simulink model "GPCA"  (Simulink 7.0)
settings: Solver=ode45  StartTime=0.0  StopTime=inf  RelTol=1e-3
PreLoadFcn:
  | GPCA_Bus_Def
InitFcn:
  | script
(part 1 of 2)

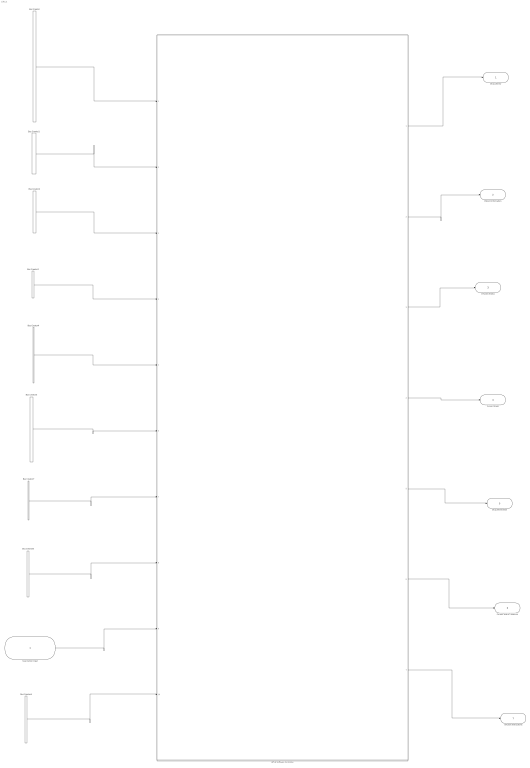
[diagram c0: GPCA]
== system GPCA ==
  User Action Input : Inport  OutDataType=sfix(16)  OutScaling=2^0
  Bus Creator : BusCreator  Tag=DrugLIibraryInput  Description=Readings from the drug library  Inputs=20  UseBusObject=on
  Bus Creator1 : BusCreator  Description=Readings from the drug library  UseBusObject=on
  Bus Creator2 : BusCreator  Inputs=6  UseBusObject=on
  Bus Creator3 : BusCreator  Inputs=3  UseBusObject=on
  Bus Creator4 : BusCreator  Inputs=12  UseBusObject=on
  Bus Creator5 : BusCreator  Inputs=11  UseBusObject=on
  Bus Creator6 : BusCreator  Inputs=2  UseBusObject=on
  Bus Creator7 : BusCreator  Inputs=3  UseBusObject=on
  Bus Creator8 : BusCreator  Inputs=3  UseBusObject=on
  GPCA Software Controller : Subsystem
  Drug Library : Outport  OutDataType=sfix(16)  OutScaling=2^0
  Patient Information : Outport  Port=2  OutDataType=sfix(16)  OutScaling=2^0
  Infusion Status : Outport  Port=3  OutDataType=sfix(16)  OutScaling=2^0
  Current State : Outport  Port=4  OutDataType=sfix(16)  OutScaling=2^0
  Drug Information : Outport  Port=5  OutDataType=sfix(16)  OutScaling=2^0
  Current Alarm Condition : Outport  Port=6  OutDataType=sfix(16)  OutScaling=2^0
  Infusion Instructions : Outport  Port=7  OutDataType=sfix(16)  OutScaling=2^0
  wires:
  Bus Creator/1 -> GPCA Software Controller/1(Drug Library Input)
  Bus Creator1/1 -> GPCA Software Controller/2(Patient Information Input)
  Bus Creator2/1 -> GPCA Software Controller/3(Drug Information Input)
  Bus Creator3/1 -> GPCA Software Controller/4(Environment Sensor Signals)
  Bus Creator4/1 -> GPCA Software Controller/5(Hardware Sensor Signals)
  Bus Creator5/1 -> GPCA Software Controller/6(Infusion Sensor Signals)
  Bus Creator7/1 -> GPCA Software Controller/7(Infusion Status Input)
  Bus Creator8/1 -> GPCA Software Controller/8(Pump Configuration Status Input)
  GPCA Software Controller/1(Drug Library Output) -> Drug Library/1
  GPCA Software Controller/2(Patient Information Output) -> Patient Information/1
  GPCA Software Controller/3(Infusion Status Output) -> Infusion Status/1
  GPCA Software Controller/4(Current State) -> Current State/1
  GPCA Software Controller/5(Drug Information Output) -> Drug Information/1
  GPCA Software Controller/6(Alarming Condition) -> Current Alarm Condition/1
  GPCA Software Controller/7(Infusion Instructions Output) -> Infusion Instructions/1
  Bus Creator6/1 -> GPCA Software Controller/10(Infusion Parameters Input)
  User Action Input/1 -> GPCA Software Controller/9(User Actions)

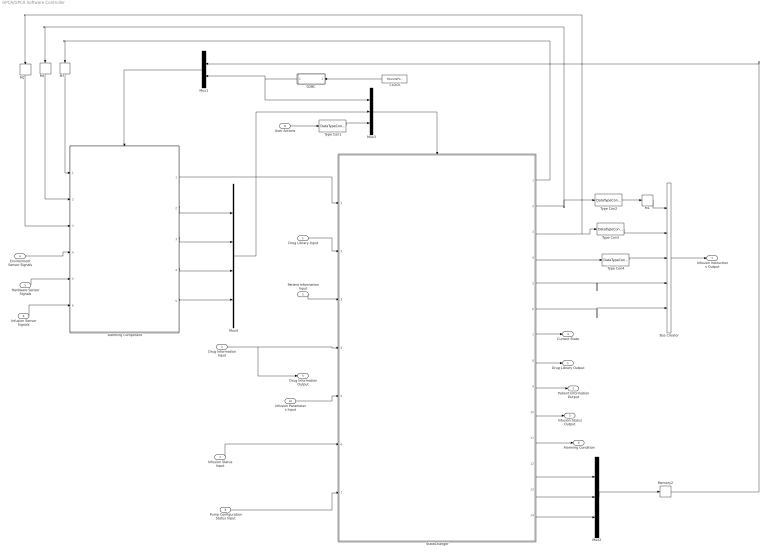
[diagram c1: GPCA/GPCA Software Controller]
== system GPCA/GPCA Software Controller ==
  Drug Library Input : Inport  OutDataType=sfix(16)  OutScaling=2^0
  Patient Information Input : Inport  Port=2  OutDataType=sfix(16)  OutScaling=2^0
  Drug Information Input : Inport  Port=3  OutDataType=sfix(16)  OutScaling=2^0
  Environment Sensor Signals : Inport  Port=4  OutDataType=sfix(16)  OutScaling=2^0
  Hardware Sensor Signals : Inport  Port=5  OutDataType=sfix(16)  OutScaling=2^0
  Infusion Sensor Signals : Inport  Port=6  OutDataType=sfix(16)  OutScaling=2^0
  Infusion Status Input : Inport  Port=7  OutDataType=sfix(16)  OutScaling=2^0
  Pump Configuration Status Input : Inport  Port=8  OutDataType=sfix(16)  OutScaling=2^0
  User Actions : Inport  Port=9  OutDataType=sfix(16)  OutScaling=2^0
  Infusion Parameters Input : Inport  Port=10  OutDataType=sfix(16)  OutScaling=2^0
  Alarming Component : Stateflow chart
  Bus Creator : BusCreator  Inputs=5  UseBusObject=on
  CLOCK : DiscretePulseGenerator  Orientation=left  PulseType=Time based  PulseWidth=50
  D2BC : Stateflow chart  Orientation=left
  M1 : Memory  InheritSampleTime=on
  M2 : Memory  Orientation=down  InheritSampleTime=on
  M4 : Memory  Orientation=down  InheritSampleTime=on
  M7 : Memory  Orientation=down  InheritSampleTime=on
  Memory2 : Memory  InheritSampleTime=on
  Mux1 : Mux  Orientation=left  Inputs=2
  Mux2 : Mux  Inputs=3
  Mux3 : Mux  Inputs=3
  Mux4 : Mux
  StateChanger : Stateflow chart
  Type Con1 : DataTypeConversion  OutDataTypeMode=boolean  OutDataType=sfix(16)  OutScaling=2^0
  Type Con2 : DataTypeConversion  OutDataType=sfix(16)  OutScaling=2^0
  Type Con3 : DataTypeConversion  OutDataType=sfix(16)  OutScaling=2^0
  Type Con4 : DataTypeConversion  OutDataType=sfix(16)  OutScaling=2^0
  Drug Library Output : Outport  OutDataType=sfix(16)  OutScaling=2^0
  Patient Information Output : Outport  Port=2  OutDataType=sfix(16)  OutScaling=2^0
  Infusion Status Output : Outport  Port=3  OutDataType=sfix(16)  OutScaling=2^0
  Current State : Outport  Port=4  OutDataType=sfix(16)  OutScaling=2^0
  Drug Information Output : Outport  Port=5  OutDataType=sfix(16)  OutScaling=2^0
  Alarming Condition : Outport  Port=6  OutDataType=sfix(16)  OutScaling=2^0
  Infusion Instructions Output : Outport  Port=7  OutDataType=sfix(16)  OutScaling=2^0
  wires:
  StateChanger/1(ClearCond) -> M7/1
  Mux3/1 -> StateChanger/Trigger
  Mux1/1 -> Alarming Component/Trigger
  StateChanger/2(O_InfusionInProgress) -> M4/1, Type Con2/1
  Alarming Component/1(ErrCond) -> StateChanger/1(ErrCond)
  User Actions/1 -> Type Con1/1
  StateChanger/12(E_Restart) -> Mux2/1
  StateChanger/13(E_AlarmClear) -> Mux2/2
  StateChanger/14(E_RequestToStart) -> Mux2/3
  Mux2/1 -> Memory2/1
  CLOCK/1 -> D2BC/1(u)
  D2BC/1(y) -> Mux1/2, Mux3/1
  Alarming Component/2(E_Alarm) -> Mux4/1
  Alarming Component/3(E_Warning) -> Mux4/2
  Alarming Component/4(E_Ready) -> Mux4/3
  Alarming Component/5(E_NotReady) -> Mux4/4
  Type Con1/1 -> Mux3/3
  Mux4/1 -> Mux3/2
  Type Con2/1 -> M1/1
  Memory2/1 -> Mux1/1
  Environment Sensor Signals/1 -> Alarming Component/4(envSenData)
  Hardware Sensor Signals/1 -> Alarming Component/5(hardwareSenData)
  Infusion Sensor Signals/1 -> Alarming Component/6(infuSenData)
  Drug Library Input/1 -> StateChanger/2(drugLibInfo)
  Patient Information Input/1 -> StateChanger/3(patientInfo)
  Drug Information Input/1 -> StateChanger/4(drugInfo), Drug Information Output/1
  Infusion Parameters Input/1 -> StateChanger/5(infuParameters)
  Infusion Status Input/1 -> StateChanger/6(infuStatus)
  Pump Configuration Status Input/1 -> StateChanger/7(pumpConfigData)
  StateChanger/11(O_AlarmCond) -> Alarming Condition/1
  StateChanger/7(O_CurrentState) -> Current State/1
  StateChanger/9(O_PatientInfo) -> Patient Information Output/1
  StateChanger/8(O_DrugLibInfo) -> Drug Library Output/1
  M1/1 -> Bus Creator/1
  StateChanger/3(O_InfusionPaused) -> M2/1, Type Con3/1
  Bus Creator/1 -> Infusion Instructions Output/1
  M7/1 -> Alarming Component/1(ClearCond)
  M4/1 -> Alarming Component/2(infusionInProgress)
  M2/1 -> Alarming Component/3(infusionPaused)
  StateChanger/4(O_BolusRequested) -> Type Con4/1
  StateChanger/5(O_ProgrammedVTBI) -> Bus Creator/4
  StateChanger/6(O_ProgrammedFlowRate) -> Bus Creator/5
  Type Con3/1 -> Bus Creator/2
  Type Con4/1 -> Bus Creator/3
  StateChanger/10(O_InfuStatus) -> Infusion Status Output/1

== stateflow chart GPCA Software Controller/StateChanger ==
  state x = displayBolusInfo [function]
    (junction 152) -> (junction 154) : [infuStatus.isBolusInProgress == 1]{bolusing := 1; ml.GAlrmMsg = MSG_BOLUSGRANT; }
    (default) -> (junction 152)
    (junction 152) -> (junction 153) : [infuStatus.isBolusInProgress == 0]{ml.GAlrmMsg = MSG_BOLUSDENIED; }
  state x1 = enterinto(stateId) [function]
    (junction 88) -> (junction 89) : {x1 := stateId;}
    (default) -> (junction 88) : {O_CurrentState := stateId;}
  state x = resumeInfusion [function]
    (junction 200) -> (junction 109) : {O_InfusionInProgress := 1;  O_InfusionPaused := 0;  O_BolusRequested := 0;}
    (default) -> (junction 199)
    (junction 199) -> (junction 200) : {infusing := 1; bolusing := 0;}
  state x = warning [function]
    (junction 127) -> (junction 108) : [ErrCond == 17]{ml.GAlrmMsg = MSG_LOWRESR;}
    (junction 127) -> (junction 128) : [ErrCond == 16]{ml.GAlrmMsg = MSG_FLOWRATEVARY;}
    (junction 127) -> (junction 115) : [ErrCond == 19]{ml.GAlrmMsg = MSG_LOGERR; }
    (junction 127) -> (junction 120) : [ErrCond == 26]{ml.GAlrmMsg = MSG_DANGERAP;}
    (junction 127) -> (junction 121) : [ErrCond ==18]{ml.GAlrmMsg = MSG_PAUSELONG;}
    (junction 127) -> (junction 122) : [ErrCond==20]{ml.GAlrmMsg = MSG_LOWBATT; }
    (junction 127) -> (junction 123) : [ErrCond==21]{ml.GAlrmMsg = MSG_WRNBATTERYCHARGE;}
    (junction 127) -> (junction 125) : [ErrCond==22]{ml.GAlrmMsg = MSG_VOLTOUTRANGE;}
    (junction 127) -> (junction 126) : [ErrCond==23]{ml.GAlrmMsg = MSG_PUMPOVERHEAT;}
    (default) -> (junction 127) : {O_AlarmCond := ErrCond;}
    (junction 127) -> (junction 131) : [ErrCond==24]{ml.GAlrmMsg = MSG_DANGERENVTEMP;}
    (junction 127) -> (junction 137) : [ErrCond == 25]{ml.GAlrmMsg = MSG_DANGERHUMD;}
  state x = initInfusion [function]
    (default) -> (junction 138)
    (junction 138) -> (junction 139) : { bolusing := 0; infusing := 0; doseRate := 0; vtbi := 0;   resetInfusionInstructions();}
  state x = checkDoseRate(iRate) [function]
    (junction 188) -> (junction 173) : [iRate <= drugLibInfo.doseRateUpperHardLimit && iRate >= drugLibInfo.doseRateLowerHardLimit]
    (junction 173) -> (junction 148) : [iRate > drugLibInfo.doseRateUpperSoftLimit || iRate < drugLibInfo.doseRateLowerSoftLimit]{ x := 1;}
    (junction 188) -> (junction 157) : [iRate > drugLibInfo.doseRateUpperHardLimit || iRate < drugLibInfo.doseRateLowerHardLimit]{ x := 2;}
    (junction 173) -> (junction 91) : [iRate <= drugLibInfo.doseRateUpperSoftLimit && iRate >= drugLibInfo.doseRateLowerSoftLimit]{ x:= 0;}
    (default) -> (junction 188)
  state x = clearAlrm (alrm) [function]
    (default) -> (junction 93) : {ClearCond := alrm;}
    (junction 93) -> (junction 94) : {E_AlarmClear;}
  state x = setPatientInfo [function]
    (default) -> (junction 167)
    (junction 167) -> (junction 169) : {O_PatientInfo.patientID := patientInfo.patientID;  O_PatientInfo.patientAge := patientInfo.patientAge;  O_PatientInfo.patientGender := patientInfo.patientGender; O_PatientInfo.patientWeight := patientInfo.patientWeight;}
  state x = initPatientInfo [function]
    (junction 187) -> (junction 144) : { O_PatientInfo.patientID := 0;  O_PatientInfo.patientAge := 0;   O_PatientInfo.patientGender := 0; O_PatientInfo.patientWeight := 0;}
    (default) -> (junction 187)
  state x = setDrugLibInfo [function]
    (junction 124) -> (junction 155) : { O_DrugLibInfo.drugConcentrationTypical = drugLibInfo.drugConcentrationTypical;   O_DrugLibInfo.drugConcentrationUpperHardLimit = drugLibInfo.drugConcentrationUpperHardLimit;   O_DrugLibInfo.drugConcentrationUpperSoftLimit = drugLibInfo.drugConcentrationUpperSoftLimit;   O_DrugLibInfo.drugConcentrationLowerSoftLimit = drugLibInfo.drugConcentrationLowerSoftLimit;   O_DrugLibInfo.drugConcentrationLowerHardLimit = drugLibInfo.drugConcentrationLowerHardLimit;}
    (default) -> (junction 132)
    (junction 132) -> (junction 143) : {O_DrugLibInfo.drugID = drugLibInfo.drugID; O_DrugLibInfo.amount = drugLibInfo.amount;}
    (junction 143) -> (junction 112) : { O_DrugLibInfo.doseRateTypical = drugLibInfo.doseRateTypical; O_DrugLibInfo.doseRateUnit = drugLibInfo.doseRateUnit;   O_DrugLibInfo.doseRateUpperHardLimit = drugLibInfo.doseRateUpperHardLimit;   O_DrugLibInfo.doseRateUpperSoftLimit = drugLibInfo.doseRateUpperSoftLimit;   O_DrugLibInfo.doseRateLowerSoftLimit = drugLibInfo.doseRateLowerSoftLimit;   O_DrugLibInfo.doseRateLowerHardLimit = drugLibInfo.doseRateLowerHardLimit;}
    (junction 112) -> (junction 124) : { O_DrugLibInfo.vtbiTypical = drugLibInfo.vtbiTypical; O_DrugLibInfo.vtbiUnit = drugLibInfo.vtbiUnit;   O_DrugLibInfo.vtbiUpperHardLimit = drugLibInfo.vtbiUpperHardLimit;   O_DrugLibInfo.vtbiUpperSoftLimit = drugLibInfo.vtbiUpperSoftLimit;   O_DrugLibInfo.vtbiLowerSoftLimit = drugLibInfo.vtbiLowerSoftLimit;   O_DrugLibInfo.vtbiLowerHardLimit = drugLibInfo.vtbiLowerHardLimit;}
  state x = setLOneMsg(fcond) [function]
    (default) -> (junction 98) : {O_AlarmCond := fcond;}
    (junction 98) -> (junction 99) : [fcond==1]{ml.GAlrmMsg =MSG_OUTOFPOWER;}
    (junction 98) -> (junction 101) : [fcond==3]{ml.GAlrmMsg = MSG_CPUFAILURE;}
    (junction 98) -> (junction 102) : [fcond==4]{ml.GAlrmMsg = MSG_MEMORYCORRUPT;}
    (junction 98) -> (junction 103) : [fcond==5]{ml.GAlrmMsg = MSG_PUMPTOOHOT;}
    (junction 98) -> (junction 104) : [fcond==6]{ml.GAlrmMsg = MSG_WATCHDOGALERT;}
    (junction 98) -> (junction 100) : [fcond==2]{ml.GAlrmMsg = MSG_REALTIMECLOCK;}
  state x = alrmLevel [function]
    (junction 96) -> (junction 184) : [ErrCond == 0]{O_AlarmCond := ErrCond; x := 0;}
    (default) -> (junction 96)
    (junction 96) -> (junction 129) : [ErrCond  > 0 && ErrCond <7] {O_AlarmCond := ErrCond; x:=1;}
    (junction 96) -> (junction 90) : [ErrCond>=7 && ErrCond < 16]{O_AlarmCond := ErrCond; x:=2;}
    (junction 96) -> (junction 97) : [ErrCond>=16]{O_AlarmCond := ErrCond; x:=3;}
  state x = setLTwoMsg(fCond) [function]
    (junction 111) -> (junction 107) : [fCond==14]{ml.GAlrmMsg = MSG_PAUSETOOLONG;}
    (junction 111) -> (junction 105) : [fCond==9]{ml.GAlrmMsg = MSG_OCCULUSION;}
    (junction 111) -> (junction 110) : [fCond==15]{ml.GAlrmMsg = MSG_AIRINLINE;}
    (default) -> (junction 111) : {O_AlarmCond := fCond;}
    (junction 111) -> (junction 113) : [fCond==7]{ml.GAlrmMsg = MSG_DOOROPEN;}
    (junction 111) -> (junction 114) : [fCond==8]{ml.GAlrmMsg = MSG_EMPTYRESERVOIR;}
    (junction 111) -> (junction 116) : [fCond==10]{ml.GAlrmMsg = MSG_OVERINFUSION;}
    (junction 111) -> (junction 117) : [fCond==11]{ml.GAlrmMsg = MSG_UNDERINFUSION;}
    (junction 111) -> (junction 118) : [fCond==12]{ml.GAlrmMsg = MSG_LESSTHANKVO;}
    (junction 111) -> (junction 119) : [fCond==13]{ml.GAlrmMsg = MSG_RATEEXCEEDCAPACITY;}
  state x = bolusStatus [function]
    (default) -> (junction 134)
    (junction 134) -> (junction 135) : [infuStatus.isBolusInProgress == 1]{bolusing := 1; ml.GAlrmMsg = MSG_BOLUSGRANT;}
    (junction 134) -> (junction 136) : [infuStatus.isBolusInProgress == 0]{bolusing := 0; ml.GAlrmMsg = MSG_BOLUSDENIED;}
  state x = checkVTBI(inputVal) [function]
    (default) -> (junction 156)
    (junction 145) -> (junction 92) : [inputVal <= drugLibInfo.vtbiUpperSoftLimit && inputVal <= drugLibInfo.vtbiLowerSoftLimit]{ x := 0;}
    (junction 145) -> (junction 95) : [inputVal > drugLibInfo.vtbiUpperSoftLimit || inputVal < drugLibInfo.vtbiLowerSoftLimit]{ x := 1;}
    (junction 156) -> (junction 146) : [inputVal > drugLibInfo.vtbiUpperHardLimit || inputVal < drugLibInfo.vtbiLowerHardLimit]{ x := 2;}
    (junction 156) -> (junction 145) : [inputVal <= drugLibInfo.vtbiUpperHardLimit && inputVal >= drugLibInfo.vtbiLowerHardLimit]
  state x = calcFlowRate(iRate) [function]
    (junction 163) -> (junction 164) : {x := iRate /  drugInfo.drugConcentration;}
    (default) -> (junction 163)
  state x = checkDrugConcentration [function]
    (junction 174) -> (junction 172) : [actualCon > upperHard || actualCon < lowerHard]{x := 2;}
    (junction 174) -> (junction 178) : [actualCon <= upperHard && actualCon >= lowerHard]
    (default) -> (junction 174) : {actualCon := drugInfo.drugConcentration; upperHard := drugLibInfo.drugConcentrationUpperHardLimit; upperSoft := drugLibInfo.drugConcentrationUpperSoftLimit; lowerHard := drugLibInfo.drugConcentrationLowerHardLimit;  lowerSoft := drugLibInfo.drugConcentrationLowerSoftLimit;}
    (junction 178) -> (junction 176) : [actualCon <= upperSoft && actualCon >= lowerSoft]{x := 0;}
    (junction 178) -> (junction 177) : [actualCon > upperSoft || actualCon < lowerSoft]{x := 1;}
  state x = initDrugLib [function]
    (junction 168) -> (junction 166) : { O_DrugLibInfo.drugID := 0; O_DrugLibInfo.amount = 0; O_DrugLibInfo.diluentVolume := 0; O_DrugLibInfo.doseRateTypical := 0;   O_DrugLibInfo.doseRateUpperHardLimit := 0; O_DrugLibInfo.doseRateUpperSoftLimit := 0; O_DrugLibInfo.doseRateLowerHardLimit := 0;   O_DrugLibInfo.doseRateLowerSoftLimit := 0; O_DrugLibInfo.doseRateUnit := 0; O_DrugLibInfo.vtbiTypical := 0; O_DrugLibInfo.vtbiUpperHardLimit := 0;   O_DrugLibInfo.vtbiUpperSoftLimit := 0; O_DrugLibInfo.vtbiLowerHardLimit := 0; O_DrugLibInfo.vtbiLowerSoftLimit := 0; O_DrugLibInfo.vtbiUnit :=0;   O_DrugLibInfo.drugConcentrationTypical := 0; O_DrugLibInfo.drugConcentrationUpperHardLimit := 0; O_DrugLibInfo.drugConcentrationUpperSoftLimit := 0;   O_DrugLibInfo.drugConcentrationLowerHardLimit := 0; O_DrugLibInfo.drugConcentrationLowerSoftLimit := 0;}
    (default) -> (junction 168)
  state x = init [function]
    (junction 159) -> (junction 130) : {temp := 0; tempx := 0; infusing :=0; bolusing :=0;}
    (default) -> (junction 183)
    (junction 183) -> (junction 159) : { ClearCond := 0; O_InfusionInProgress := 0; O_InfusionPaused := 0;   O_BolusRequested := 0; O_ProgrammedVTBI := 0; O_ProgrammedFlowRate := 0; O_CurrentState := 0;   O_AlarmCond := 0;  initDrugLib(); initPatientInfo();}
  state InfusionStateMachine
    state ConfirmPowerDown
      en: enterinto(2);
      ml.GMsgConStr := MSG_POWEROFF;
    state PowerOff
      en: enterinto(1);
      ex: ml.GMsgConStr = MSG_WELCOME;
    state POST
      en: enterinto(3);
      tempx := pumpConfigData.isPOSTSuccessful ;
    state ALM_POSTFailed
      en:  ml.GMsgConStr =MSG_POSTFAIL;
      enterinto(4);
    state InfusionInSession
      state InfusionPaused
        en: enterinto(36);
        pauseInfusion();
        ml.GMsgConStr = MSG_INFUSIONPAUSED;
      state PausedStopConfirm
        en: ml.GMsgConStr = MSG_SPCHOOSE;
        enterinto(38);
      state InfusionStopped
        en: copyInfuStatus();
        stopInfusion();
        ml.GMsgConStr = MSG_INFUSIONSTOP;
        enterinto(39);
      state EmptyReservoir
        en: enterinto(40);
        ml.GAlrmMsg = MSG_EMPTYRESERVOIR;
      state CheckDrugWhileInfusing
        en: ml.GMsgConStr = MSG_CHECKTYPE
        enterinto(41);
        tempx := checkDrug();
      state ALMWrongDrug
        en: ml.GMsgConStr = MSG_WRONGDRUG;
        enterinto(42);
      state LevelTwoAlarming
        en: enterinto(44);
        setLTwoMsg(ErrCond);
      state InfusionSubMachine
        state Infusing
          en:  ml.GMsgConStr = MSG_INFUSING;
          enterinto(28);
          copyInfuStatus();
          on every(3, E_Clock):
          copyInfuStatus();
        state ChangeRate
          en: ml.GMsgConStr = MSG_CHANGEDR;
          ml.GSetConVal =temp;
          enterinto(30);
          copyInfuStatus();
          on every(3, E_Clock):
          copyInfuStatus();
        state CheckNewRate
          en: ml.GMsgConStr = MSG_CHECKDR;
          tempx = checkDoseRate(infuParameters.programmedDoseRate);
          temp = infuParameters.programmedDoseRate;
          enterinto(31);
          copyInfuStatus();
          on every(3, E_Clock):
          copyInfuStatus();
        state ALM_NewRateOutBound
          en: ml.GMsgConStr = MSG_ALRMDR ;
          enterinto(32);
          copyInfuStatus();
          on every(3, E_Clock):
          copyInfuStatus();
        state ConfirmStop
          en: ml.GMsgConStr = MSG_CONFIRMSTOP;
          enterinto(35);
          copyInfuStatus();
          on every(3, E_Clock):
          copyInfuStatus();
        state ConfirmPause
          en: ml.GMsgConStr = MSG_CONFIRMPAUSE;
          enterinto(34);
          copyInfuStatus();
          on every(3, E_Clock):
          copyInfuStatus();
        state BolusRequest
          en: enterinto(29);
        Infusing -> ConfirmPause : E_PauseInfusion
        Infusing -> ChangeRate : E_ChangeDoseRate
        ChangeRate -> Infusing : E_Cancel
        ChangeRate -> CheckNewRate : E_ConfirmDoseRate
        CheckNewRate -> ALM_NewRateOutBound : [tempx>0]
        CheckNewRate -> Infusing : [tempx==0]{setDoseRate(temp); O_ProgrammedFlowRate := calcFlowRate(temp);}
        ALM_NewRateOutBound -> Infusing : E_Cancel
        (default) -> Infusing
        ConfirmPause -> Infusing : E_Cancel
        ConfirmStop -> Infusing : E_Cancel
        (junction 149) -> Infusing : [infuStatus.isBolusInProgress == 1]{ml.GAlrmMsg = MSG_BOLUSDENIED;}
        Infusing -> (junction 149) : E_RequestBolus
        ConfirmPause -> InfusionSubMachine : E_ConfirmPauseInfusion{ml.GAlrmMsg = MSG_BLANK;}
        Infusing -> InfusionSubMachine : [infusionDone(vtbi) == 1] {ml.GAlrmMsg = MSG_BLANK;}
        Infusing -> ConfirmStop : E_StopInfusion
        ConfirmStop -> InfusionSubMachine : E_ConfirmStopInfusion{ml.GAlrmMsg = MSG_BLANK;}
        ALM_NewRateOutBound -> ChangeRate : E_ChangeDoseRate
        ChangeRate -> ChangeRate : E_Warning{warning();}
        ALM_NewRateOutBound -> ALM_NewRateOutBound : E_Warning{warning();}
        ConfirmStop -> ConfirmStop : E_Warning{warning();}
        Infusing -> Infusing : E_Warning{warning();}
        ConfirmPause -> ConfirmPause : E_Warning{warning();}
        InfusionSubMachine -> Infusing : E_Ready {startInfusion();}
        BolusRequest -> (junction 133) : {O_BolusRequested := 0;}
        (junction 133) -> Infusing : {displayBolusInfo();}
        (junction 149) -> BolusRequest : [infuStatus.isBolusInProgress == 0]{O_BolusRequested := 1;}
        Infusing -> Infusing : [infusing > 0 && bolusing > 0 && infuStatus.isBolusInProgress == 0]{bolusing :=0; ml.GAlrmMsg = MSG_STOPBOLUS;}
        InfusionSubMachine -> Infusing : E_Cancel{resumeInfusion();}
        InfusionSubMachine -> Infusing : [tempx == 0]{resumeInfusion();}
        InfusionSubMachine -> Infusing : E_ClearAlarm{clearLevel2Alarm(); resumeInfusion();}
        InfusionSubMachine -> Infusing : E_ClearAlarm{ClearCond:=13; resumeInfusion();E_AlarmClear}
        ChangeRate -> Infusing : [infusionDone(vtbi) == 1]
        ALM_NewRateOutBound -> Infusing : [infusionDone(vtbi) == 1]
        ConfirmStop -> Infusing : [infusionDone(vtbi) == 1]
        ConfirmPause -> Infusing : [infusionDone(vtbi) == 1]
        ConfirmPause -> ConfirmPause : [infusing > 0 && bolusing > 0 && infuStatus.isBolusInProgress == 0]{bolusing :=0; ml.GAlrmMsg = MSG_STOPBOLUS;}
        ConfirmStop -> ConfirmStop : [infusing > 0 && bolusing > 0 && infuStatus.isBolusInProgress == 0] {bolusing :=0; ml.GAlrmMsg = MSG_STOPBOLUS;}
        ChangeRate -> ChangeRate : [infusing > 0 && bolusing > 0 && infuStatus.isBolusInProgress == 0] {bolusing :=0; ml.GAlrmMsg = MSG_STOPBOLUS;}
        ALM_NewRateOutBound -> ALM_NewRateOutBound : [infusing > 0 && bolusing > 0 && infuStatus.isBolusInProgress == 0] {bolusing :=0; ml.GAlrmMsg = MSG_STOPBOLUS;}
      state PausedTooLong
        en: enterinto(37);
        ml.GAlrmMsg = MSG_PAUSETOOLONG;
      InfusionPaused -> LevelTwoAlarming : [alrmLevel()==2]{pauseInfusion();}
      InfusionInSession -> InfusionSubMachine : E_Ready {startInfusion();}
      InfusionStopped -> InfusionInSession : E_NewInfusion{resetInfusionInstructions(); initInfuStatus();}
      InfusionPaused -> InfusionSubMachine : E_Cancel{resumeInfusion();}
      InfusionPaused -> PausedTooLong : E_Alarm[ErrCond == 13]
      PausedTooLong -> InfusionSubMachine : E_ClearAlarm{ClearCond:=13; resumeInfusion();E_AlarmClear}
      InfusionPaused -> PausedStopConfirm : E_StopInfusion
      PausedStopConfirm -> InfusionPaused : E_Cancel
      PausedStopConfirm -> InfusionStopped : E_ConfirmStopInfusion
      EmptyReservoir -> CheckDrugWhileInfusing : E_CheckDrug
      CheckDrugWhileInfusing -> InfusionSubMachine : [tempx == 0]{resumeInfusion();}
      CheckDrugWhileInfusing -> ALMWrongDrug : [tempx > 0]
      EmptyReservoir -> InfusionStopped : E_StopInfusion
      ALMWrongDrug -> InfusionStopped : E_StopInfusion
      LevelTwoAlarming -> EmptyReservoir : [ErrCond==7]
      (default) -> InfusionSubMachine
      InfusionSubMachine -> LevelTwoAlarming : [alrmLevel()==2]{pauseInfusion();}
      LevelTwoAlarming -> InfusionStopped : E_StopInfusion{clearLevel2Alarm();}
      ALMWrongDrug -> ALMWrongDrug : E_Warning{warning();}
      PausedStopConfirm -> LevelTwoAlarming : [alrmLevel()==2]{pauseInfusion();}
      ALMWrongDrug -> CheckDrugWhileInfusing : E_CheckDrug
      LevelTwoAlarming -> LevelTwoAlarming : E_Warning{warning();}
      EmptyReservoir -> EmptyReservoir : E_Warning{warning();}
      InfusionStopped -> InfusionStopped : E_Warning{warning();}
      InfusionPaused -> InfusionPaused : E_Warning{warning();}
      PausedStopConfirm -> PausedStopConfirm : E_Warning{warning();}
      PausedTooLong -> PausedTooLong : E_Warning{warning();}
      LevelTwoAlarming -> InfusionSubMachine : E_ClearAlarm{clearLevel2Alarm(); resumeInfusion();}
      PausedTooLong -> InfusionStopped : E_StopInfusion
      InfusionSubMachine -> InfusionStopped : [infusionDone(vtbi) == 1] {ml.GAlrmMsg = MSG_BLANK;}
      Infusing -> InfusionStopped : [infusionDone(vtbi) == 1] {ml.GAlrmMsg = MSG_BLANK;}
      InfusionPaused -> Infusing : E_Cancel{resumeInfusion();}
      CheckDrugWhileInfusing -> Infusing : [tempx == 0]{resumeInfusion();}
      LevelTwoAlarming -> Infusing : E_ClearAlarm{clearLevel2Alarm(); resumeInfusion();}
      PausedTooLong -> Infusing : E_ClearAlarm{ClearCond:=13; resumeInfusion();E_AlarmClear}
      InfusionSubMachine -> InfusionStopped : E_ConfirmStopInfusion{ml.GAlrmMsg = MSG_BLANK;}
      ConfirmStop -> InfusionStopped : E_ConfirmStopInfusion{ml.GAlrmMsg = MSG_BLANK;}
      InfusionSubMachine -> InfusionPaused : E_ConfirmPauseInfusion{ml.GAlrmMsg = MSG_BLANK;}
      ConfirmPause -> InfusionPaused : E_ConfirmPauseInfusion{ml.GAlrmMsg = MSG_BLANK;}
    state Init
    state POSTDONE
      en: ml.GMsgConStr = MSG_POSTDONE;
      enterinto(45);
      tempx = 0;
    state LEVELONEALRM
      en: setLOneMsg(ErrCond);
      enterinto(43);
    state CheckDrugRoutine
      state CheckAdminSet
        en: enterinto(5);
        ml.GMsgConStr =MSG_ADMINCHECK;
        tempx := pumpConfigData.isAdminSetCheckPassed;
      state CheckPrime
        en:  enterinto(7);
        tempx = 0;
        ml.GMsgConStr = MSG_PRIME;
        tempx = pumpConfigData.isPumpPrimed;
      state ALM_WrongAdminCheck
        en: enterinto(6);
        ml.GMsgConStr = MSG_ADMINFAIL;
      state PrimeFailed
        en: enterinto(8);
        ml.GMsgConStr = MSG_PRIMEFAIL;
      state DisplayDrugInfo
        en: enterinto(9);
        tempx = 0;
        ml.GMsgConStr = MSG_DRUGINFO;
      state CheckDrug_CheckType
        en: enterinto(10);
        ml.GMsgConStr = MSG_CHECKTYPE;
        tempx := checkDrugType();
      state UnknownDrug
        en: enterinto(11);
        ml.GMsgConStr =MSG_WRONGDRUG;
      state Check_DrugUnits
        en: enterinto(12);
        ml.GMsgConStr = MSG_CHECKDU;
        tempx := checkDrugUnits();
      state IncorrectDrugUnits
        en: enterinto(13);
        ml.GMsgConStr =MSG_WRONGDU;
      state Check_Concen
        en:enterinto(14);
        ml.GMsgConStr = MSG_CHECKCON;
        tempx := checkDrugConcentration();
      state WrongConcentration
        en: enterinto(15);
        ml.GMsgConStr = MSG_WRONGCON;
      state WRN_DangerCon
        en: enterinto(16);
        ml.GMsgConStr = MSG_DANGECON;
      state DisplayPatientProfile
        en:   enterinto(18);
        ml.GMsgConStr = MSG_PATIENTINFO;
      UnknownDrug -> CheckDrug_CheckType : E_CheckDrug
      Check_Concen -> WrongConcentration : [tempx==2]
      Check_DrugUnits -> IncorrectDrugUnits : [tempx!=0]
      IncorrectDrugUnits -> CheckDrug_CheckType : E_CheckDrug
      Check_DrugUnits -> Check_Concen : [tempx==0]
      CheckDrug_CheckType -> UnknownDrug : [tempx==1]
      CheckDrug_CheckType -> Check_DrugUnits : [tempx==0]
      Check_Concen -> WRN_DangerCon : [tempx==1]
      Check_Concen -> DisplayPatientProfile : [tempx==0]{setPatientInfo();}
      WRN_DangerCon -> DisplayPatientProfile : E_ConfirmConcentration{setPatientInfo();}
      DisplayPatientProfile -> CheckDrugRoutine : E_ConfigureInfusionProgram{setDrugLibInfo();}
      ALM_WrongAdminCheck -> CheckAdminSet : E_CheckAdminSet
      CheckAdminSet -> ALM_WrongAdminCheck : [tempx==0]
      CheckAdminSet -> CheckPrime : [tempx==1]{E_Restart; }
      PrimeFailed -> CheckPrime : E_Prime
      CheckPrime -> PrimeFailed : [tempx==0]
      CheckPrime -> DisplayDrugInfo : [tempx==1]{setDrugLibInfo();}
      DisplayPatientProfile -> DisplayDrugInfo : E_Cancel
      DisplayDrugInfo -> CheckDrug_CheckType : E_CheckDrug
      ALM_WrongAdminCheck -> ALM_WrongAdminCheck : E_Warning{warning();}
      UnknownDrug -> UnknownDrug : E_Warning{warning();}
      WrongConcentration -> CheckDrug_CheckType : E_CheckDrug
      WrongConcentration -> WrongConcentration : E_Warning{warning();}
      CheckDrugRoutine -> CheckAdminSet : E_NewInfusion{resetInfusionInstructions(); initInfuStatus();}
      CheckDrugRoutine -> CheckAdminSet : E_CheckAdminSet{resetInfusionInstructions(); initInfuStatus();}
      DisplayDrugInfo -> DisplayDrugInfo : E_Warning{warning();}
      WRN_DangerCon -> WRN_DangerCon : E_Warning{warning();}
      WRN_DangerCon -> CheckDrug_CheckType : E_CheckDrug
      DisplayPatientProfile -> DisplayPatientProfile : E_Warning{warning();}
      PrimeFailed -> PrimeFailed : E_Warning{warning();}
      IncorrectDrugUnits -> IncorrectDrugUnits : E_Warning{warning();}
    state ConfigureInfusionProgram
      state ALM_VTBIOutBound
        en: enterinto(22);
        ml.GMsgConStr = MSG_ALMVTBI;
      state DisplayDoseRate
        en:  enterinto(23);
        ml.GMsgConStr = MSG_DISPLAYDR;
        tempx = 0;
        setDoseRate(drugLibInfo.doseRateTypical);
      state DisplayVTBI
        en:   enterinto(19);
        ml.GMsgConStr = MSG_VTBI;
        setVTBI(drugLibInfo.vtbiTypical);
      state ChangeVTBI
        en: enterinto(20);
        ml.GMsgConStr = MSG_CHANGEVTBI;
      state CheckVTBI
        en: enterinto(21);
        ml.GMsgConStr = MSG_CHECKVTBI;
        tempx := checkVTBI(infuParameters.programmedVTBI);
      state ChangeDoseRate
        en: enterinto(24);
        ml.GMsgConStr = MSG_CHANGEDR;
      state CheckDoseRate
        en: enterinto(25);
        ml.GMsgConStr = MSG_CHECKDR;
        tempx := checkDoseRate(infuParameters.programmedDoseRate);
      state ALM_DoseRateOutBound
        en: enterinto(26);
        ml.GMsgConStr = MSG_ALRMDR;
      state DisplaySettings
        en: enterinto(27);
        ml.GMsgConStr = MSG_DISPLAYSET;
      state ReadyToStart
        en: enterinto(48);
      state WRN_VTBIOutBound
        en: enterinto(46);
        ml.GMsgConStr = MSG_WRNVTBI;
      state WRN_DOSERATEOUTSOFTLIMITS
        en:  enterinto(47);
        ml.GMsgConStr = MSG_WRNDR;
      CheckVTBI -> ALM_VTBIOutBound : [tempx==2]
      ALM_VTBIOutBound -> ChangeVTBI : E_ChangeVTBI
      CheckVTBI -> DisplayDoseRate : [tempx==0]{setVTBI(infuParameters.programmedVTBI);}
      ChangeVTBI -> CheckVTBI : E_ConfirmVTBI
      DisplayVTBI -> ChangeVTBI : E_ChangeVTBI
      ChangeVTBI -> DisplayVTBI : E_Cancel
      DisplayVTBI -> DisplayDoseRate : E_ConfirmVTBI
      DisplayDoseRate -> ChangeDoseRate : E_ChangeDoseRate
      ChangeDoseRate -> DisplayDoseRate : E_Cancel
      ChangeDoseRate -> CheckDoseRate : E_ConfirmDoseRate
      CheckDoseRate -> ALM_DoseRateOutBound : [tempx==2]
      ALM_DoseRateOutBound -> ChangeDoseRate : E_ChangeDoseRate
      CheckDoseRate -> DisplaySettings : [tempx==0]{setDoseRate(infuParameters.programmedDoseRate);}
      DisplayDoseRate -> DisplaySettings : E_ConfirmDoseRate
      DisplaySettings -> ReadyToStart : E_StartInfusion{E_RequestToStart}
      DisplaySettings -> DisplaySettings : E_Warning{warning();}
      WRN_VTBIOutBound -> WRN_VTBIOutBound : E_Warning{warning();}
      ReadyToStart -> ReadyToStart : E_Warning{warning();}
      DisplayVTBI -> DisplayVTBI : E_Warning{warning();}
      ReadyToStart -> DisplaySettings : E_NotReady{ml.GAlrmMsg = MSG_NOTREADY;}
      DisplaySettings -> DisplayVTBI : E_ConfigureInfusionProgram
      ChangeDoseRate -> ChangeDoseRate : E_Warning{warning();}
      ReadyToStart -> ConfigureInfusionProgram : E_Ready {startInfusion();}
      CheckVTBI -> WRN_VTBIOutBound : [tempx==1]
      WRN_VTBIOutBound -> DisplayDoseRate : E_ConfirmVTBI{setVTBI(infuParameters.programmedVTBI);}
      WRN_VTBIOutBound -> ChangeVTBI : E_ChangeVTBI
      ConfigureInfusionProgram -> DisplayVTBI : E_ConfigureInfusionProgram{setDrugLibInfo();}
      WRN_DOSERATEOUTSOFTLIMITS -> DisplaySettings : E_ConfirmDoseRate{setDoseRate(infuParameters.programmedDoseRate);}
      CheckDoseRate -> WRN_DOSERATEOUTSOFTLIMITS : [tempx==1]
      DisplayDoseRate -> DisplayDoseRate : E_Warning{warning();}
      ALM_DoseRateOutBound -> ALM_DoseRateOutBound : E_Warning{warning();}
      ALM_VTBIOutBound -> ALM_VTBIOutBound : E_Warning{warning();}
      ChangeVTBI -> ChangeVTBI : E_Warning{warning();}
      WRN_DOSERATEOUTSOFTLIMITS -> ChangeDoseRate : E_ChangeDoseRate
    Init -> PowerOff
    ALM_POSTFailed -> PowerOff : E_PowerButton
    PowerOff -> POST : E_PowerButton{init(); ml.GMsgConStr = MSG_POST;}
    ConfirmPowerDown -> CheckDrugRoutine : E_Cancel[tempx==1]
    InfusionInSession -> ConfirmPowerDown : E_PowerButton{tempx=3;}
    POSTDONE -> POSTDONE : E_Warning{warning();}
    ConfirmPowerDown -> PowerOff : E_ConfirmPowerDown{O_AlarmCond := 0; ml.GAlrmMsg := MSG_BLANK;}
    ConfirmPowerDown -> ConfigureInfusionProgram : E_Cancel[tempx==2]
    ConfigureInfusionProgram -> ConfirmPowerDown : E_PowerButton{tempx=2;}
    ConfirmPowerDown -> InfusionInSession : E_Cancel[tempx==3]
    InfusionInSession -> LEVELONEALRM : [alrmLevel()==1]{resetInfusionInstructions();}
    InfusionStopped -> CheckAdminSet : E_NewInfusion{resetInfusionInstructions(); initInfuStatus();}
    POSTDONE -> CheckAdminSet : E_CheckAdminSet{resetInfusionInstructions(); initInfuStatus();}
    ConfirmPowerDown -> ConfirmPowerDown : E_Warning{warning();}
    ALM_POSTFailed -> ALM_POSTFailed : E_Warning{warning();}
    POST -> ALM_POSTFailed : [tempx==0]
    CheckDrugRoutine -> LEVELONEALRM : [alrmLevel()==1]
    (default) -> Init
    ConfigureInfusionProgram -> LEVELONEALRM : [alrmLevel()==1]
    LEVELONEALRM -> PowerOff : E_PowerButton {O_AlarmCond := 0; ml.GAlrmMsg := MSG_BLANK;}
    POSTDONE -> ConfirmPowerDown : E_PowerButton{tempx=4;}
    ConfirmPowerDown -> POSTDONE : E_Cancel[tempx==4]
    POST -> POSTDONE : [tempx==1]
    POSTDONE -> CheckDrugRoutine : E_CheckAdminSet{resetInfusionInstructions(); initInfuStatus();}
    DisplayPatientProfile -> DisplayVTBI : E_ConfigureInfusionProgram{setDrugLibInfo();}
    ConfigureInfusionProgram -> InfusionInSession : E_Ready {startInfusion();}
    ReadyToStart -> Infusing : E_Ready {startInfusion();}
    InfusionInSession -> CheckDrugRoutine : E_NewInfusion{resetInfusionInstructions(); initInfuStatus();}
    CheckDrugRoutine -> ConfirmPowerDown : E_PowerButton{tempx=1;}
    CheckDrugRoutine -> ConfigureInfusionProgram : E_ConfigureInfusionProgram{setDrugLibInfo();}
  state x = infusionDone(expectedVolume) [function]
    (default) -> (junction 106) : {x:=0;}
    (junction 106) -> (junction 141) : [infuStatus.totalVolumeInfused < expectedVolume]{x := 0;}
    (junction 106) -> (junction 142) : [infuStatus.totalVolumeInfused >= expectedVolume]{x := 1;}
  state x = clearLevel2Alarm [function]
    (junction 185) -> (junction 186) : {ml.GAlrmMsg = MSG_BLANK; E_AlarmClear;}
    (default) -> (junction 185)
  state x = checkDrugType [function]
    (junction 181) -> (junction 175) : [drugInfo.drugDoseAmount == drugLibInfo.amount]{x := 0;}
    (junction 181) -> (junction 171) : [drugInfo.drugDoseAmount != drugLibInfo.amount]{x := 1;}
    (default) -> (junction 182)
    (junction 182) -> (junction 147) : [drugInfo.drugID != drugLibInfo.drugID]{x:=1;}
    (junction 182) -> (junction 181) : [drugInfo.drugID == drugLibInfo.drugID]
  state x = checkDrug [function]
    (junction 162) -> (junction 161) : [flag == 1]{x := 1;}
    (default) -> (junction 162) : {flag := checkDrugType();}
    (junction 192) -> (junction 140) : [flag == 1]{x := 1;}
    (junction 192) -> (junction 189) : [flag == 0]{flag:= checkDrugConcentration();}
    (junction 189) -> (junction 191) : [flag == 0]{x := 0;}
    (junction 189) -> (junction 190) : [flag > 0]{x := 1;}
    (junction 162) -> (junction 192) : [flag == 0]{flag := checkDrugUnits();}
  state x = checkDrugUnits [function]
    (junction 150) -> (junction 158) : [drugInfo.drugVolumeUnit == drugLibInfo.vtbiUnit]{ x:= 0;}
    (default) -> (junction 170)
    (junction 150) -> (junction 160) : [drugInfo.drugVolumeUnit != drugLibInfo.vtbiUnit]{x := 1;}
    (junction 170) -> (junction 150) : [drugInfo.drugDoseUnit == drugLibInfo.doseRateUnit]
    (junction 170) -> (junction 151) : [drugInfo.drugDoseUnit != drugLibInfo.doseRateUnit]{x := 1;}
  state x = stopInfusion [function]
    (junction 194) -> (junction 193) : {O_ProgrammedVTBI := 0;  O_ProgrammedFlowRate := 0;}
    (junction 209) -> (junction 194) : {O_InfusionInProgress := 0;  O_InfusionPaused := 0;  O_BolusRequested := 0;}
    (default) -> (junction 208)
    (junction 208) -> (junction 209) : {infusing := 0; bolusing := 0;}
  state x = setVTBI(iVTBI) [function]
    (default) -> (junction 195)
    (junction 195) -> (junction 196) : {vtbi := iVTBI;}
  state x = setDoseRate(iRate) [function]
    (default) -> (junction 197)
    (junction 197) -> (junction 198) : {doseRate := iRate;}
  state x = startInfusion [function]
    (default) -> (junction 201)
    (junction 201) -> (junction 202) : {O_ProgrammedFlowRate := calcFlowRate(doseRate);  O_ProgrammedVTBI := vtbi;}
    (junction 202) -> (junction 203) : {O_InfusionInProgress := 1;  O_InfusionPaused := 0;  O_BolusRequested := 0;}
    (junction 203) -> (junction 204) : {infusing := 1; bolusing := 0;}
  state x = pauseInfusion [function]
    (default) -> (junction 205)
    (junction 205) -> (junction 206) : {infusing := 0; bolusing := 0;}
    (junction 206) -> (junction 207) : {O_InfusionInProgress := 1;  O_InfusionPaused := 1;  O_BolusRequested := 0;}
  state x = resetInfusionInstructions [function]
    (junction 211) -> (junction 210) : {stopInfusion();}
    (default) -> (junction 211)
  state x = copyInfuStatus [function]
    (default) -> (junction 212)
    (junction 212) -> (junction 213) : {O_InfuStatus.isBolusInProgress := infuStatus.isBolusInProgress;  O_InfuStatus.totalVolumeInfused := infuStatus.totalVolumeInfused;  O_InfuStatus.remainingVolumeInReservoir := infuStatus.remainingVolumeInReservoir;}
  state x = initInfuStatus [function]
    (default) -> (junction 214)
    (junction 214) -> (junction 215) : {O_InfuStatus.isBolusInProgress := 0;  O_InfuStatus.totalVolumeInfused := 0;  O_InfuStatus.remainingVolumeInReservoir := infuStatus.remainingVolumeInReservoir;}
  state x = outputInfuStatus(a,b,c) [function]
    (default) -> (junction 216)
    (junction 216) -> (junction 217) : {O_InfuStatus.isBolusInProgress := a;  O_InfuStatus.totalVolumeInfused := b;  O_InfuStatus.remainingVolumeInReservoir := c;}
